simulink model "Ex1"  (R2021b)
settings: Solver=VariableStepAuto  StartTime=0.0  StopTime=10.0  RelTol=1e-3  AbsTol=1e-3
libraries: fl_lib x35, nesl_utility x9

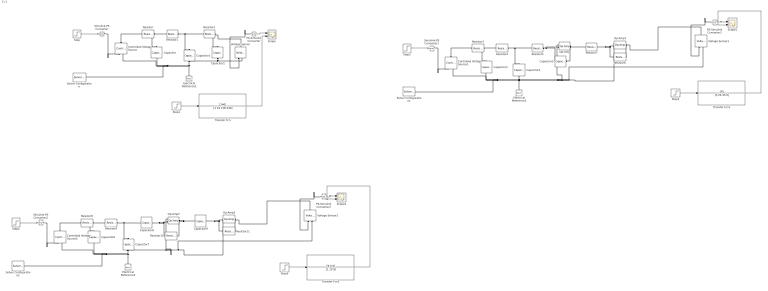
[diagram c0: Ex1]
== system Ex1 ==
  Capacitor : fl_lib/Electrical/Electrical Elements/Capacitor  c=2 uF  r=0 Ohm  g=0 1/Ohm  i_specify=off  i_priority=None  i=0 A  i_nominal_specify=off  i_nominal_unit=A  i_nominal_value=1  v_specify=off  v_priority=None  v=0 V  v_nominal_specify=off  v_nominal_unit=V  v_nominal_value=1  vc_specify=off  vc_priority=High  vc=0 V  vc_nominal_specify=off  vc_nominal_unit=V  vc_nominal_value=1
  Capacitor1 : fl_lib/Electrical/Electrical Elements/Capacitor  c=10/6 uF  r=0 Ohm  g=0 1/Ohm  i_specify=off  i_priority=None  i=0 A  i_nominal_specify=off  i_nominal_unit=A  i_nominal_value=1  v_specify=off  v_priority=None  v=0 V  v_nominal_specify=off  v_nominal_unit=V  v_nominal_value=1  vc_specify=off  vc_priority=High  vc=0 V  vc_nominal_specify=off  vc_nominal_unit=V  vc_nominal_value=1
  Capacitor2 : fl_lib/Electrical/Electrical Elements/Capacitor  c=10/8 uF  r=0 Ohm  g=0 1/Ohm  i_specify=off  i_priority=None  i=0 A  i_nominal_specify=off  i_nominal_unit=A  i_nominal_value=1  v_specify=off  v_priority=None  v=0 V  v_nominal_specify=off  v_nominal_unit=V  v_nominal_value=1  vc_specify=off  vc_priority=High  vc=0 V  vc_nominal_specify=off  vc_nominal_unit=V  vc_nominal_value=1
  Capacitor3 : fl_lib/Electrical/Electrical Elements/Capacitor  c=2 uF  r=0 Ohm  g=0 1/Ohm  i_specify=off  i_priority=None  i=0 A  i_nominal_specify=off  i_nominal_unit=A  i_nominal_value=1  v_specify=off  v_priority=None  v=0 V  v_nominal_specify=off  v_nominal_unit=V  v_nominal_value=1  vc_specify=off  vc_priority=High  vc=0 V  vc_nominal_specify=off  vc_nominal_unit=V  vc_nominal_value=1
  Capacitor4 : fl_lib/Electrical/Electrical Elements/Capacitor  c=10/3 uF  r=0 Ohm  g=0 1/Ohm  i_specify=off  i_priority=None  i=0 A  i_nominal_specify=off  i_nominal_unit=A  i_nominal_value=1  v_specify=off  v_priority=None  v=0 V  v_nominal_specify=off  v_nominal_unit=V  v_nominal_value=1  vc_specify=off  vc_priority=High  vc=0 V  vc_nominal_specify=off  vc_nominal_unit=V  vc_nominal_value=1
  Capacitor{5,7..9} (4 alike) : fl_lib/Electrical/Electrical Elements/Capacitor  c=10 uF  r=0 Ohm  g=0 1/Ohm  i_specify=off  i_priority=None  i=0 A  i_nominal_specify=off  i_nominal_unit=A  i_nominal_value=1  v_specify=off  v_priority=None  v=0 V  v_nominal_specify=off  v_nominal_unit=V  v_nominal_value=1  vc_specify=off  vc_priority=High  vc=0 V  vc_nominal_specify=off  vc_nominal_unit=V  vc_nominal_value=1
  Capacitor6 : fl_lib/Electrical/Electrical Elements/Capacitor  c=10/9 uF  r=0 Ohm  g=0 1/Ohm  i_specify=off  i_priority=None  i=0 A  i_nominal_specify=off  i_nominal_unit=A  i_nominal_value=1  v_specify=off  v_priority=None  v=0 V  v_nominal_specify=off  v_nominal_unit=V  v_nominal_value=1  vc_specify=off  vc_priority=High  vc=0 V  vc_nominal_specify=off  vc_nominal_unit=V  vc_nominal_value=1
  Controlled Voltage Source : fl_lib/Electrical/Electrical Sources/Controlled Voltage Source
  Controlled Voltage Source1 : fl_lib/Electrical/Electrical Sources/Controlled Voltage Source
  Controlled Voltage Source2 : fl_lib/Electrical/Electrical Sources/Controlled Voltage Source
  Electrical Reference1 : fl_lib/Electrical/Electrical Elements/Electrical Reference
  Electrical Reference2 : fl_lib/Electrical/Electrical Elements/Electrical Reference
  Electrical Reference3 : fl_lib/Electrical/Electrical Elements/Electrical Reference
  Op-Amp{,1..3} (4 alike) : fl_lib/Electrical/Electrical Elements/Op-Amp  outI_specify=off  outI_priority=None  outI=0 A  outI_nominal_specify=off  outI_nominal_unit=A  outI_nominal_value=1
  PS-Simulink Converter : nesl_utility/PS-Simulink Converter  PhysicalDomain=network_engine_domain  SubClassName=ps_output  LeftPortType=input  RightPortType=output  PseudoPeriodic=off  Frequencies=[]  Unit=inherit  AffineConversion=off
  PS-Simulink Converter1 : nesl_utility/PS-Simulink Converter  PhysicalDomain=network_engine_domain  SubClassName=ps_output  LeftPortType=input  RightPortType=output  PseudoPeriodic=off  Frequencies=[]  Unit=inherit  AffineConversion=off
  PS-Simulink Converter2 : nesl_utility/PS-Simulink Converter  PhysicalDomain=network_engine_domain  SubClassName=ps_output  LeftPortType=input  RightPortType=output  PseudoPeriodic=off  Frequencies=[]  Unit=inherit  AffineConversion=off
  Resistor{,1..5,8..11} (10 alike) : fl_lib/Electrical/Electrical Elements/Resistor  R=100000 Ohm  i_specify=off  i_priority=None  i=0 A  i_nominal_specify=off  i_nominal_unit=A  i_nominal_value=1  v_specify=off  v_priority=None  v=0 V  v_nominal_specify=off  v_nominal_unit=V  v_nominal_value=1
  Resistor6 : fl_lib/Electrical/Electrical Elements/Resistor  R=8000 Ohm  i_specify=off  i_priority=None  i=0 A  i_nominal_specify=off  i_nominal_unit=A  i_nominal_value=1  v_specify=off  v_priority=None  v=0 V  v_nominal_specify=off  v_nominal_unit=V  v_nominal_value=1
  Resistor7 : fl_lib/Electrical/Electrical Elements/Resistor  R=45000 Ohm  i_specify=off  i_priority=None  i=0 A  i_nominal_specify=off  i_nominal_unit=A  i_nominal_value=1  v_specify=off  v_priority=None  v=0 V  v_nominal_specify=off  v_nominal_unit=V  v_nominal_value=1
  Scope : Scope  NumInputPorts=2
  Scope1 : Scope  NumInputPorts=2
  Scope2 : Scope  NumInputPorts=2
  Simulink-PS Converter : nesl_utility/Simulink-PS Converter  PhysicalDomain=network_engine_domain  SubClassName=ps_input  LeftPortType=input  RightPortType=output  PseudoPeriodic=off  Frequencies=[]  NoiseDistribution=none  NoiseParameters=[]  Unit=1  AffineConversion=off  FilteringAndDerivatives=provide  SimscapeFilterOrder=1  InputFilterTimeConstant=0.001  UdotUserProvided=0
  Simulink-PS Converter1 : nesl_utility/Simulink-PS Converter  PhysicalDomain=network_engine_domain  SubClassName=ps_input  LeftPortType=input  RightPortType=output  PseudoPeriodic=off  Frequencies=[]  NoiseDistribution=none  NoiseParameters=[]  Unit=1  AffineConversion=off  FilteringAndDerivatives=provide  SimscapeFilterOrder=1  InputFilterTimeConstant=0.001  UdotUserProvided=0
  Simulink-PS Converter2 : nesl_utility/Simulink-PS Converter  PhysicalDomain=network_engine_domain  SubClassName=ps_input  LeftPortType=input  RightPortType=output  PseudoPeriodic=off  Frequencies=[]  NoiseDistribution=none  NoiseParameters=[]  Unit=1  AffineConversion=off  FilteringAndDerivatives=provide  SimscapeFilterOrder=1  InputFilterTimeConstant=0.001  UdotUserProvided=0
  Solver Configuration : nesl_utility/Solver Configuration  PhysicalDomain=network_engine_domain  SubClassName=solver  LeftPortType=input  RightPortType=generic  Tones=[]  Harmonics=[]  SimulateNoise=off  Profile=off  UseLocalSampling=off  EnableSwitchedLinearOptims=on  FrequencyDomain=off  UseCCode=off  RelTol=0.001  AbsTol=1e-06  MinStep=1e-09  ToWorkspace=off  RevertToSquareIcSolve=off  NumHomotopyIterations=100  PhasorMode=off  PhasorModeNumHarmonics=1  DoDC=off  ResidualTolerance=1e-09  UseLocalSolver=off  LocalSolverChoice=NE_BACKWARD_EULER_ADVANCER  LocalSolverSampleTime=0.001  DoFixedCost=off  MaxNonlinIter=3  MaxModeIter=2  ComputeImpulses=off  ImpulseIterations=2  LinearAlgebra=auto  EquationFormulation=NE_TIME_EF  DelaysMemoryBudget=1024  AutomaticFiltering=on  FilteringTimeConstant=0.001  PartitionStorageMethod=AS_NEEDED  PartitionMemoryBudget=1024  PartitionMethod=ROBUST
  Solver Configuration1 : nesl_utility/Solver Configuration  PhysicalDomain=network_engine_domain  SubClassName=solver  LeftPortType=input  RightPortType=generic  Tones=[]  Harmonics=[]  SimulateNoise=off  Profile=off  UseLocalSampling=off  EnableSwitchedLinearOptims=on  FrequencyDomain=off  UseCCode=off  RelTol=0.001  AbsTol=1e-06  MinStep=1e-09  ToWorkspace=off  RevertToSquareIcSolve=off  NumHomotopyIterations=100  PhasorMode=off  PhasorModeNumHarmonics=1  DoDC=off  ResidualTolerance=1e-09  UseLocalSolver=off  LocalSolverChoice=NE_BACKWARD_EULER_ADVANCER  LocalSolverSampleTime=0.001  DoFixedCost=off  MaxNonlinIter=3  MaxModeIter=2  ComputeImpulses=off  ImpulseIterations=2  LinearAlgebra=auto  EquationFormulation=NE_TIME_EF  DelaysMemoryBudget=1024  AutomaticFiltering=on  FilteringTimeConstant=0.001  PartitionStorageMethod=AS_NEEDED  PartitionMemoryBudget=1024  PartitionMethod=ROBUST
  Solver Configuration2 : nesl_utility/Solver Configuration  PhysicalDomain=network_engine_domain  SubClassName=solver  LeftPortType=input  RightPortType=generic  Tones=[]  Harmonics=[]  SimulateNoise=off  Profile=off  UseLocalSampling=off  EnableSwitchedLinearOptims=on  FrequencyDomain=off  UseCCode=off  RelTol=0.001  AbsTol=1e-06  MinStep=1e-09  ToWorkspace=off  RevertToSquareIcSolve=off  NumHomotopyIterations=100  PhasorMode=off  PhasorModeNumHarmonics=1  DoDC=off  ResidualTolerance=1e-09  UseLocalSolver=off  LocalSolverChoice=NE_BACKWARD_EULER_ADVANCER  LocalSolverSampleTime=0.001  DoFixedCost=off  MaxNonlinIter=3  MaxModeIter=2  ComputeImpulses=off  ImpulseIterations=2  LinearAlgebra=auto  EquationFormulation=NE_TIME_EF  DelaysMemoryBudget=1024  AutomaticFiltering=on  FilteringTimeConstant=0.001  PartitionStorageMethod=AS_NEEDED  PartitionMemoryBudget=1024  PartitionMethod=ROBUST
  Step : Step  SampleTime=0
  Step1 : Step  SampleTime=0
  Step{2..5} (4 alike) : Step  Time=0  SampleTime=0
  Transfer Fcn : TransferFcn  Numerator=[240]  Denominator=[1 19 118 240]
  Transfer Fcn1 : TransferFcn  Numerator=[8]  Denominator=[3 24 45 0]
  Transfer Fcn2 : TransferFcn  Numerator=[9 0 0]  Denominator=[1 10 9]
  Voltage Sensor : fl_lib/Electrical/Electrical Sensors/Voltage Sensor
  Voltage Sensor1 : fl_lib/Electrical/Electrical Sensors/Voltage Sensor
  Voltage Sensor2 : fl_lib/Electrical/Electrical Sensors/Voltage Sensor
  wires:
  PS-Simulink Converter/1 -> Scope/1
  Step/1 -> Simulink-PS Converter/1
  Transfer Fcn/1 -> Scope/2
  Step1/1 -> Transfer Fcn/1
  Transfer Fcn1/1 -> Scope1/2
  Step3/1 -> Transfer Fcn1/1
  Step2/1 -> Simulink-PS Converter1/1
  PS-Simulink Converter1/1 -> Scope1/1
  Transfer Fcn2/1 -> Scope2/2
  Step4/1 -> Simulink-PS Converter2/1
  Step5/1 -> Transfer Fcn2/1
  PS-Simulink Converter2/1 -> Scope2/1
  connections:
  Resistor/RConn1 -- Capacitor/LConn1 -- Resistor1/LConn1
  Resistor1/RConn1 -- Resistor2/LConn1 -- Capacitor1/LConn1
  Resistor2/RConn1 -- Voltage Sensor/LConn1 -- Capacitor2/LConn1
  Capacitor2/RConn1 -- Voltage Sensor/RConn2 -- Solver Configuration/RConn1 -- Controlled Voltage Source/RConn2 -- Capacitor/RConn1 -- Electrical Reference1/LConn1 -- Capacitor1/RConn1
  Voltage Sensor/RConn1 -- PS-Simulink Converter/LConn1
  Simulink-PS Converter/RConn1 -- Controlled Voltage Source/RConn1
  Controlled Voltage Source/LConn1 -- Resistor/LConn1
  Capacitor4/RConn1 -- Op-Amp/LConn1 -- Op-Amp1/LConn1 -- Voltage Sensor1/RConn2 -- Solver Configuration1/RConn1 -- Controlled Voltage Source1/RConn2 -- Capacitor3/RConn1 -- Electrical Reference2/LConn1
  Resistor4/RConn1 -- Capacitor4/LConn1 -- Resistor5/LConn1
  Resistor3/RConn1 -- Capacitor3/LConn1 -- Resistor4/LConn1
  Controlled Voltage Source1/LConn1 -- Resistor3/LConn1
  Simulink-PS Converter1/RConn1 -- Controlled Voltage Source1/RConn1
  Voltage Sensor1/RConn1 -- PS-Simulink Converter1/LConn1
  Resistor5/RConn1 -- Capacitor5/LConn1 -- Op-Amp/LConn2
  Capacitor5/RConn1 -- Resistor7/LConn1 -- Op-Amp/RConn1
  Op-Amp1/LConn2 -- Resistor7/RConn1 -- Resistor6/LConn1
  Resistor6/RConn1 -- Voltage Sensor1/LConn1 -- Op-Amp1/RConn1
  Op-Amp2/RConn1 -- Capacitor9/LConn1 -- Resistor10/RConn1
  Voltage Sensor2/RConn2 -- Op-Amp3/LConn1 -- Op-Amp2/LConn1 -- Controlled Voltage Source2/RConn2 -- Capacitor6/RConn1 -- Solver Configuration2/RConn1 -- Electrical Reference3/LConn1 -- Capacitor7/RConn1
  Op-Amp3/LConn2 -- Capacitor9/RConn1 -- Resistor11/LConn1
  Resistor8/RConn1 -- Capacitor6/LConn1 -- Resistor9/LConn1
  Resistor11/RConn1 -- Voltage Sensor2/LConn1 -- Op-Amp3/RConn1
  Op-Amp2/LConn2 -- Capacitor8/RConn1 -- Resistor10/LConn1
  Resistor9/RConn1 -- Capacitor8/LConn1 -- Capacitor7/LConn1
  Controlled Voltage Source2/LConn1 -- Resistor8/LConn1
  Voltage Sensor2/RConn1 -- PS-Simulink Converter2/LConn1
  Simulink-PS Converter2/RConn1 -- Controlled Voltage Source2/RConn1
